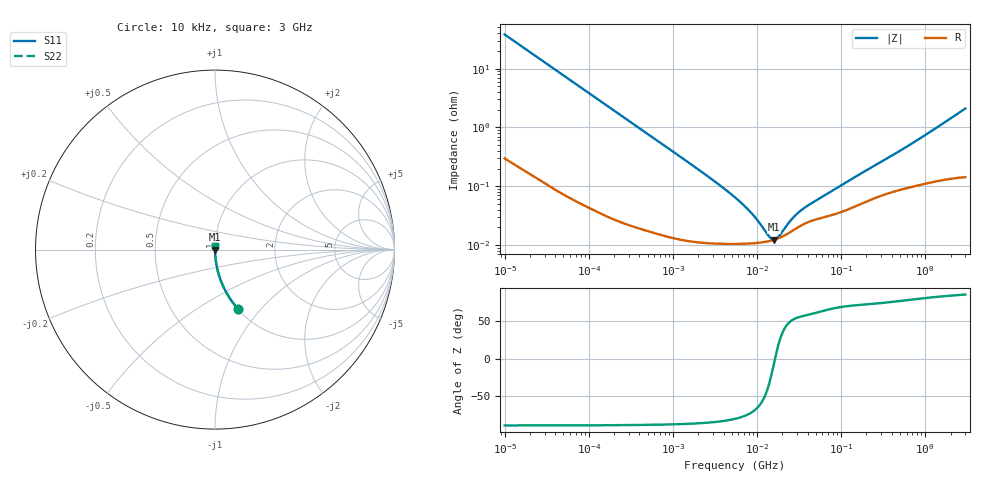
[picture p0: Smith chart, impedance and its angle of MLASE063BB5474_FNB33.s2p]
! MLASE063BB5474_FNB33  S-PARAMETER MODEL  ( Standard Model )
! Model Generated by TAIYO YUDEN Corporation (http://www.ty-top.com)
! Version 2.0
! TAIYO YUDEN Control No. 241120
! Copyright(c) 2017 TAIYO YUDEN CO.,LTD. All Rights Reserved.
! Product Description (link to TY-COMPAS)
! https://ds.yuden.co.jp/TYCOMPAS/or/detail?pn=MLASE063BB5474KFNB33&u=M
! Products Name : Multilayer Ceramic Capacitors
! Characteristics :
!  Capacitance : 0.47 [uF] , Rated Voltage : 16 [V] , TCC : X5R
!  Case Size : 0.6 x 0.3 / 0.024 x 0.012 [mm/inch] , Thickness : 0.3 / 0.012 [mm/inch]
!  (Conditions: Temperature = 25 [degC] , DC Bias Voltage = 0 [V])
! External Node Assignments :
!  1  o---| |---o  2
! GND o---------o GND
! Frequency Range : 10kHz  -  3GHz  [ 401 STEP ]
# MHZ S RI R 50
! Freq[MHz].  S11 Real  S11 Imag  S21 Real  S21 Imag  S12 Real  S12 Imag  S22 Real  S22 Imag
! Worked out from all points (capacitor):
!   401 points, 10 kHz to 3 GHz, reference 50 ohm
!   read as one part in series: C = 418 nF near 10.65 kHz
!   lowest |Z| = 12.3 mohm at 16 MHz (marker M1)
!   series resonance near 16.37 MHz, so ESL is about 230 pH
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0.01  0.1284 -0.3307  0.8716 0.3307  0.8716 0.3307  0.1284 -0.3307
0.015549  0.0584 -0.2304  0.9416 0.2304  0.9416 0.2304  0.0584 -0.2304
0.026575  0.0215 -0.1406  0.9785 0.1406  0.9785 0.1406  0.0215 -0.1406
0.045421  0.00784 -0.0837  0.9922 0.0837  0.9922 0.0837  0.00784 -0.0837
0.082683  0.00265 -0.0464  0.9974 0.0464  0.9974 0.0464  0.00265 -0.0464
0.683653  0.000184 -0.00569  0.9998 0.00569  0.9998 0.00569  0.000184 -0.00569
2.652321  0.000109 -0.00144  0.9999 0.00144  0.9999 0.00144  0.000109 -0.00144
5.477226  0.000105 -0.000637  0.9999 0.000637  0.9999 0.000637  0.000105 -0.000637
7.048603  0.000105 -0.000455  0.9999 0.000455  0.9999 0.000455  0.000105 -0.000455
8.789267  0.000107 -0.000319  0.9999 0.000319  0.9999 0.000319  0.000107 -0.000319
14.10408  0.000117 -7.19e-05  0.9999 7.19e-05  0.9999 7.19e-05  0.000117 -7.19e-05
15.02209  0.00012 -4.14e-05  0.9999 4.14e-05  0.9999 4.14e-05  0.00012 -4.14e-05
15.99985  0.000123 -1.1e-05  0.9999 1.1e-05  0.9999 1.1e-05  0.000123 -1.1e-05
17.04125  0.000126 1.92e-05  0.9999 -1.92e-05  0.9999 -1.92e-05  0.000126 1.92e-05
18.15044  0.000131 4.92e-05  0.9999 -4.92e-05  0.9999 -4.92e-05  0.000131 4.92e-05
24.10585  0.000161 0.000182  0.9998 -0.000182  0.9998 -0.000182  0.000161 0.000182
29.12589  0.000191 0.000267  0.9998 -0.000267  0.9998 -0.000267  0.000191 0.000267
35.19136  0.000223 0.000346  0.9998 -0.000346  0.9998 -0.000346  0.000223 0.000346
45.28751  0.00026 0.000453  0.9997 -0.000453  0.9997 -0.000453  0.00026 0.000453
374.4521  0.000775 0.00303  0.9992 -0.00303  0.9992 -0.00303  0.000775 0.00303
823.6  0.00107 0.00611  0.9989 -0.00611  0.9989 -0.00611  0.00107 0.00611
3000  0.00186 0.0209  0.9981 -0.0209  0.9981 -0.0209  0.00186 0.0209
